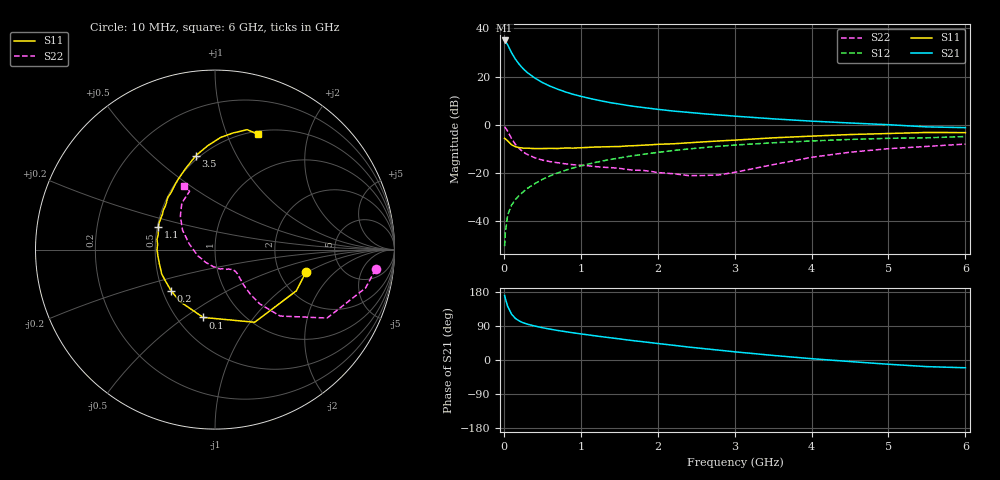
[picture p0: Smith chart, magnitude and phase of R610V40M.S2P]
! SIEMENS Small Signal Semiconductors
! BFR193
! Si NPN RF Bipolar Junction Transistor in SOT23
! VCE = 10 V  IC = 40 mA
! Common Emitter S-Parameters:  May  1996
# GHz  S  MA  R  50
!  f  S11  S21  S12  S22
! GHz  MAG  ANG  MAG  ANG  MAG  ANG  MAG  ANG
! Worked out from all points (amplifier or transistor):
!   36 points, 10 MHz to 6 GHz, reference 50 ohm
!   highest |S21| = 35.0 dB at 10 MHz (marker M1)
!   |S21| within 3 dB of that: start of sweep to 68.05 MHz
!   unconditionally stable (mu >= 1): 473.3 MHz to 2.22 GHz
!   at 250 MHz: K = 0.91, MSG = 25.6 dB, |S12| = -28.0 dB
!   at 1.4 GHz: K = 1.02, MAG = 10.8 dB, |S12| = -14.4 dB
!   at 6 GHz: K = 0.94, MSG = 1.8 dB, |S12| = -4.9 dB
!   S11 on the Smith chart (normalised r, x): 10 MHz: 2.83, -0.96; 100 MHz: 0.67, -0.59; 200 MHz: 0.55, -0.29; 1.1 GHz: 0.51, +0.14; 3.5 GHz: 0.48, +0.70; 6 GHz: 0.54, +1.30
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0.01  0.5229 -13.6  56.4 170.3  0.003 73.4  0.9017 -7.0
0.02  0.5081 -26.9  54.41 161.9  0.0058 72.5  0.8656 -14.3
0.05  0.461 -61.4  45.62 141.5  0.0134 67.8  0.7318 -31.4
0.1  0.3836 -99.8  31.54 121.1  0.0213 65.2  0.518 -45.6
0.15  0.3495 -123.9  23.09 109.7  0.0279 65.2  0.3912 -50.5
0.2  0.3351 -136.9  18.02 103.1  0.0341 67.3  0.3201 -51.6
0.25  0.327 -147.1  14.66 98.3  0.04 68.4  0.273 -51.3
0.3  0.3265 -155.4  12.33 94.9  0.0469 69.7  0.2437 -50.6
0.4  0.3196 -166.5  9.412 89.7  0.0595 71.0  0.2067 -48.8
0.5  0.32 -173.7  7.557 85.3  0.073 71.7  0.1843 -47.2
0.6  0.323 179.7  6.341 81.5  0.0866 71.2  0.1714 -46.8
0.8  0.3286 169.9  4.81 74.8  0.1132 69.8  0.1539 -47.7
0.9  0.3268 165.9  4.296 71.8  0.1267 68.8  0.1478 -48.0
1.1  0.3388 158.5  3.574 66.2  0.1529 66.7  0.1399 -52.1
1.3  0.3472 151.0  3.057 60.8  0.1791 64.2  0.1306 -56.1
1.6  0.3625 142.4  2.53 53.1  0.2171 60.3  0.118 -66.1
2.2  0.402 127.3  1.928 39.0  0.2908 51.6  0.0961 -95.3
2.8  0.4608 113.6  1.596 25.9  0.3577 42.7  0.0908 -146.1
3.5  0.5346 101.5  1.326 12.1  0.4219 31.9  0.1483 167.0
4.5  0.6258 87.1  1.087 -4.1  0.4953 18.1  0.2689 135.9
5.5  0.6917 75.0  0.902 -17.5  0.5355 4.6  0.3549 113.5
6  0.6856 69.3  0.871 -20.5  0.569 0.8  0.3967 116.0
